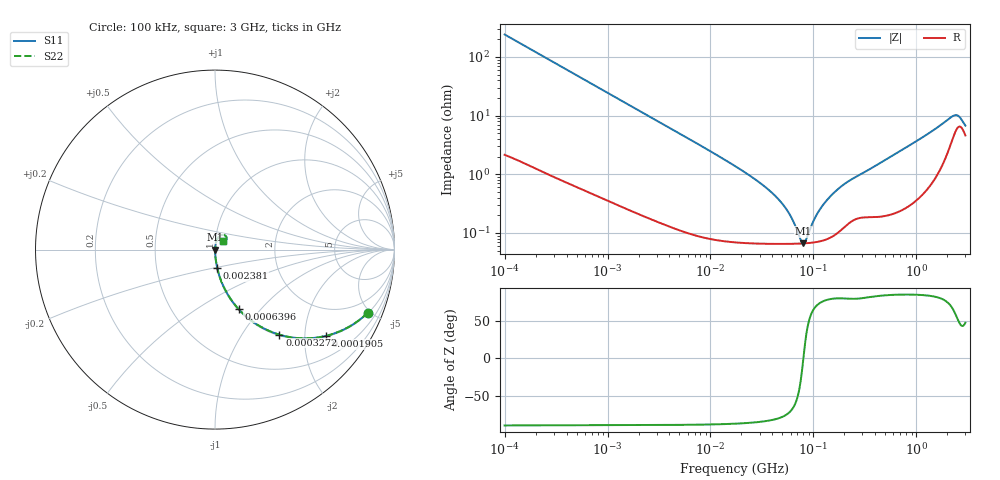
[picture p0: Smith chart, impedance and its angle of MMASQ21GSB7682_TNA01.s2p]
! MMASQ21GSB7682_TNA01  S-PARAMETER MODEL  ( Standard Model )
! Model Generated by TAIYO YUDEN Corporation (http://www.ty-top.com)
! Version 1.0
! TAIYO YUDEN Control No. 220601
! Copyright(c) 2013 TAIYO YUDEN CO.,LTD. All Rights Reserved.
! Product Description (link to TY-COMPAS)
! https://ds.yuden.co.jp/TYCOMPAS/or/detail?pn=MMASQ21GSB7682KTNA01&u=M
! Products Name : Multilayer Ceramic Capacitors
! Characteristics :
!  Capacitance : 6800 [pF] , Rated Voltage : 250 [V] , TCC : X7R
!  Case Size : 2.0 x 1.25 / 0.079 x 0.049 [mm/inch] , Thickness : 1.25 / 0.049 [mm/inch]
!  (Conditions: Temperature = 25 [degC] , DC Bias Voltage = 0 [V])
! External Node Assignments :
!  1  o---| |---o  2
! GND o---------o GND
! Frequency Range : 100kHz  -  3GHz  [ 401 STEP ]
# MHZ S RI R 50
! Freq[MHz].  S11 Real  S11 Imag  S21 Real  S21 Imag  S12 Real  S12 Imag  S22 Real  S22 Imag
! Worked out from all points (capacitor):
!   401 points, 100 kHz to 3 GHz, reference 50 ohm
!   read as one part in series: C = 6.56 nF near 105.3 kHz
!   lowest |Z| = 66.4 mohm at 79.24 MHz (marker M1)
!   series resonance near 79.99 MHz, so ESL is about 600 pH
!   S11 on the Smith chart (normalised r, x): 100 kHz: 1.04, -4.84; 190.5 kHz: 1.03, -2.55; 327.2 kHz: 1.02, -1.49; 639.6 kHz: 1.01, -0.77; 2.381 MHz: 1.00, -0.21; 3 GHz: 1.09, +0.10
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0.1  0.852 -0.3507  0.148 0.3507  0.148 0.3507  0.852 -0.3507
0.190467  0.6184 -0.4807  0.3816 0.4807  0.3816 0.4807  0.6184 -0.4807
0.327242  0.3587 -0.474  0.6413 0.474  0.6413 0.474  0.3587 -0.474
0.562235  0.1626 -0.3627  0.8374 0.3627  0.8374 0.3627  0.1626 -0.3627
0.639561  0.1313 -0.3312  0.8687 0.3312  0.8687 0.3312  0.1313 -0.3312
1.09883  0.0506 -0.212  0.9494 0.212  0.9494 0.212  0.0506 -0.212
2.380755  0.0125 -0.1025  0.9875 0.1025  0.9875 0.1025  0.0125 -0.1025
3.161081  0.0076 -0.0778  0.9924 0.0778  0.9924 0.0778  0.0076 -0.0778
17.7727  0.000866 -0.0134  0.9991 0.0134  0.9991 0.0134  0.000866 -0.0134
32.15051  0.000696 -0.00654  0.9993 0.00654  0.9993 0.00654  0.000696 -0.00654
47.32384  0.00066 -0.00345  0.9993 0.00345  0.9993 0.00345  0.00066 -0.00345
59.67813  0.000654 -0.00187  0.9993 0.00187  0.9993 0.00187  0.000654 -0.00187
75.25761  0.000658 -0.000385  0.9993 0.000385  0.9993 0.000385  0.000658 -0.000385
79.23846  0.000661 -5.94e-05  0.9993 5.94e-05  0.9993 5.94e-05  0.000661 -5.94e-05
85.60801  0.000667 0.00043  0.9993 -0.00043  0.9993 -0.00043  0.000667 0.00043
97.38194  0.000683 0.00126  0.9993 -0.00126  0.9993 -0.00126  0.000683 0.00126
122.8043  0.000744 0.00282  0.9993 -0.00282  0.9993 -0.00282  0.000744 0.00282
171.6802  0.00102 0.0054  0.999 -0.0054  0.999 -0.0054  0.00102 0.0054
547.5153  0.00238 0.0191  0.9976 -0.0191  0.9976 -0.0191  0.00238 0.0191
2259.438  0.0458 0.0819  0.9542 -0.0819  0.9542 -0.0819  0.0458 0.0819
2570.185  0.065 0.0658  0.935 -0.0658  0.935 -0.0658  0.065 0.0658
3000  0.0461 0.0452  0.9539 -0.0452  0.9539 -0.0452  0.0461 0.0452
